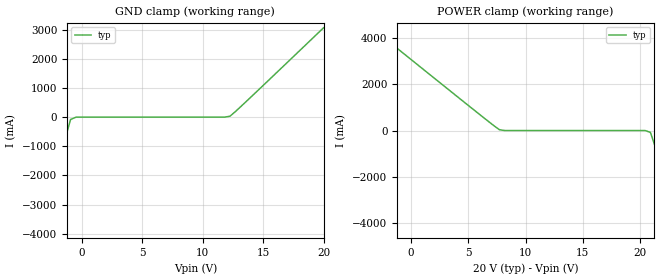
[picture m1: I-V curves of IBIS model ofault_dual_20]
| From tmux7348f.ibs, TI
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| ofault_dual_20
[Model]   ofault_dual_20
Model_type   Input
Vinl = 0.8
Vinh = 1.3
|   typ   min   max
C_comp   2.533030e-12   NA   NA
[Voltage Range]   20   NA   NA
[Temperature Range]   27   NA   NA
[Power Clamp Reference]   20   NA   NA
[GND Clamp Reference]   0   NA   NA
[GND Clamp]
|   Voltage   I(typ)   I(min)   I(max)
-25V      -323.5A    NA         NA
-2.727V   -4.807A    NA         NA
-2.273V   -2.271A    NA         NA
-1.364V   -746.5mA   NA         NA
-909.1mV  -80.83mA   NA         NA
-454.5mV  -314uA     NA         NA
11.82V    32.4nA     NA         NA
12.27V    33.31mA    NA         NA
20V       3.067A     NA         NA
[POWER Clamp]
|   Voltage   I(typ)   I(min)   I(max)
-5V       5.056A     NA         NA
-3.636V   4.513A     NA         NA
-3.182V   4.332A     NA         NA
7.727V    33.31mA    NA         NA
8.182V    32.4nA     NA         NA
20.45V    -314uA     NA         NA
20.91V    -80.83mA   NA         NA
21.36V    -746.5mA   NA         NA
22.27V    -2.271A    NA         NA
22.73V    -4.807A    NA         NA
40V       -251.7A    NA         NA
